VAR_GLOBAL CONSTANT
	
	cOversamples   : UDINT := 1;    		 // oversampling of I/O Terminal
	cBufferLength  : UDINT := 1200;   		 // Size of buffer transfered to RMS functionblock
	cRMSBuffer     : UDINT := 3600;  		 // e.g. keep 2 old buffers in mind and add one new buffer to calc RMS value
	cChannels      : UDINT := 1;		     // amount of channels to process in RMS functionblock
END_VAR
